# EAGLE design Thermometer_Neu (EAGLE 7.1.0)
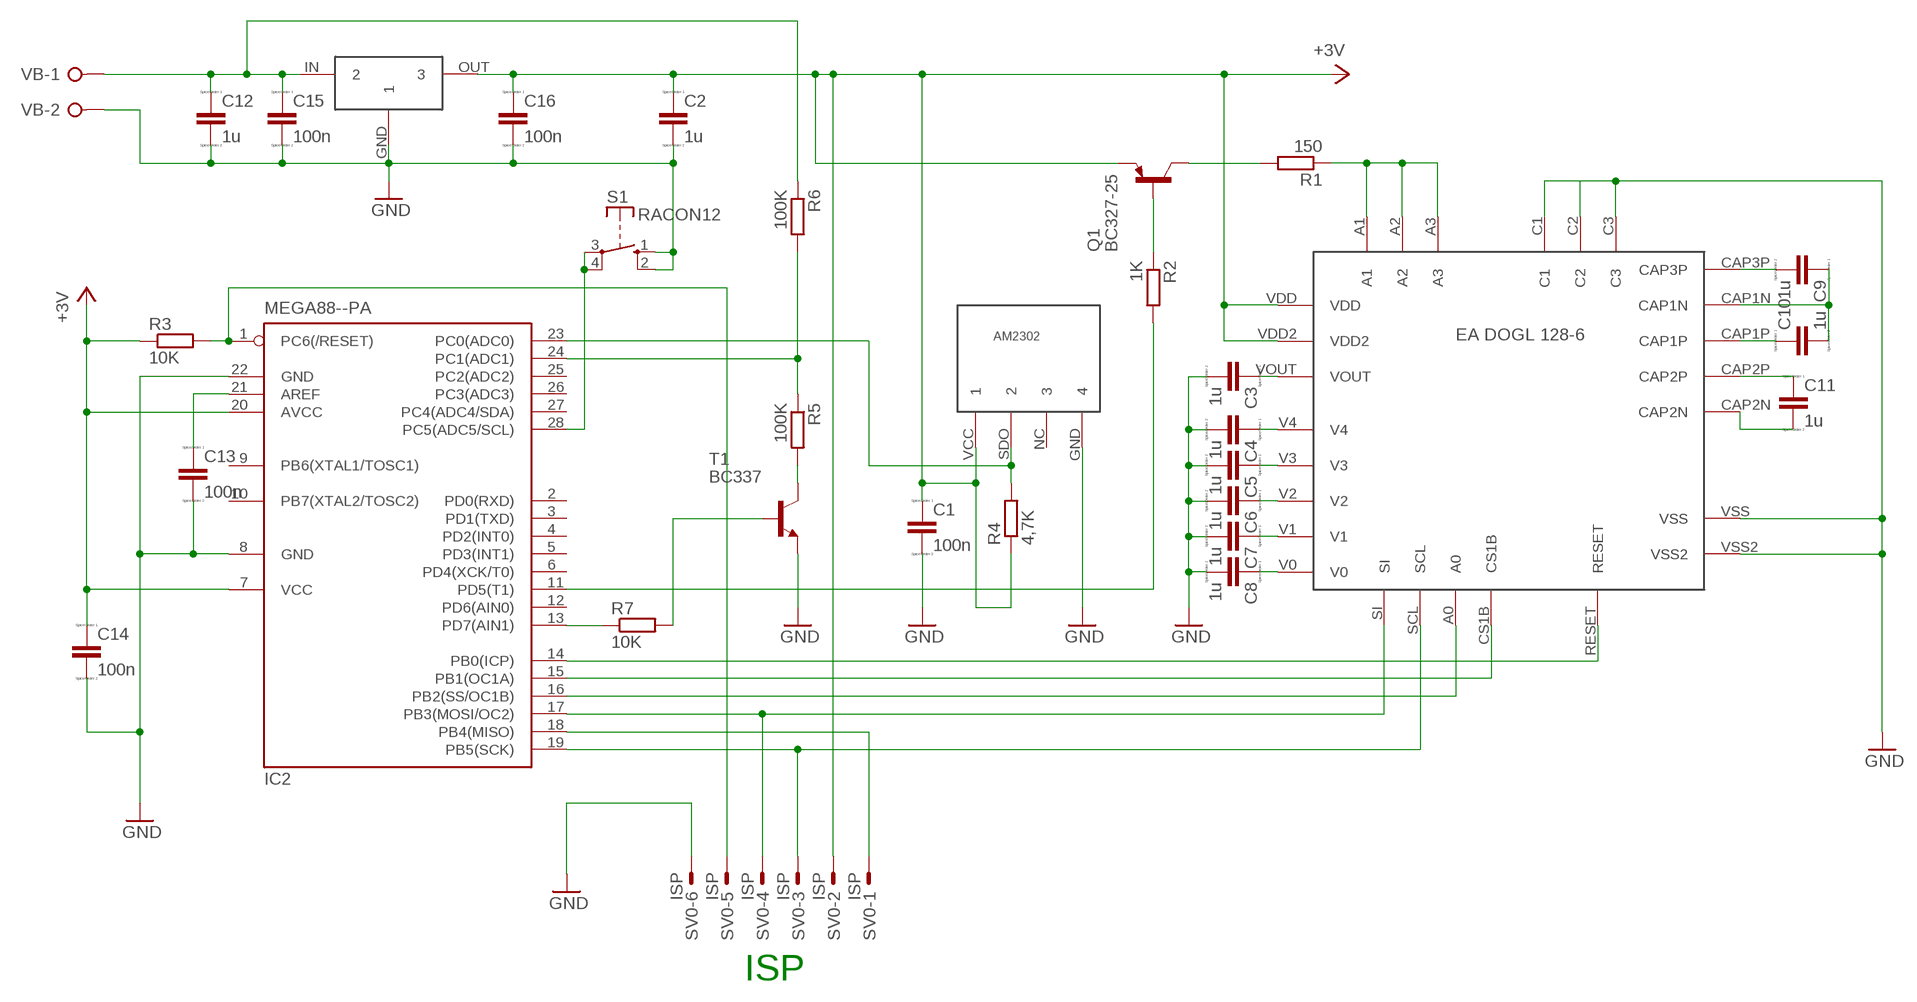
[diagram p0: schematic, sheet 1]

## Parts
C1  100n  C-EUC1206K  [C1206K]
C2  1u  C-EUC1206K  [C1206K]
C3  1u  C-EUC1206K  [C1206K]
C4  1u  C-EUC1206K  [C1206K]
C5  1u  C-EUC1206K  [C1206K]
C6  1u  C-EUC1206K  [C1206K]
C7  1u  C-EUC1206K  [C1206K]
C8  1u  C-EUC1206K  [C1206K]
C9  1u  C-EUC1206K  [C1206K]
C10  1u  C-EUC1206K  [C1206K]
C11  1u  C-EUC1206K  [C1206K]
C12  1u  C-EUC1206K  [C1206K]
C13  100n  C-EUC1206K  [C1206K]
C14  100n  C-EUC1206K  [C1206K]
C15  100n  C-EUC1206K  [C1206K]
C16  100n  C-EUC1206K  [C1206K]
IC2  MEGA88--PA  MEGA8-P  [DIL28-3]
Q1  BC327-25  [TO92-EBC]
R1  150  R-EU_0207/15  [0207/15]
R2  1K  R-EU_0207/15  [0207/15]
R3  10K  R-EU_0207/15  [0207/15]
R4  4,7K  R-EU_0207/15  [0207/15]
R5  100K  R-EU_0207/15  [0207/15]
R6  100K  R-EU_0207/15  [0207/15]
R7  10K  R-EU_0207/15  [0207/15]
S1  RACON12  [RACON12]
SV0  ISP  ML6E  [ML6]
T1  BC337  [TO92]
U$1  LDO  [LDO]
U$2  AM2302  [AM2302]
U$3  EA_DOGL_128_6  [EA_DOGL_128-6]
VB  W237-02P  [W237-132]

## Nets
+3V3: C1.1 C2.1 C14.1 C16.1 IC2.7(VCC) IC2.20(AVCC) Q1.E R3.1 R4.1 SV0.2 U$1.OUT U$2.VCC U$3.VDD U$3.VDD2 ; supply symbol labelled +3V
GND: C1.2 C2.2 C3.2 C4.2 C5.2 C6.2 C7.2 C8.2 C12.2 C13.2 C14.2 C15.2 C16.2 IC2.8(GND) IC2.22(GND) S1.1(S) S1.2(S) SV0.6 T1.1(E) U$1.GND U$2.GND U$3.C1 U$3.C2 U$3.C3 U$3.VSS U$3.VSS2 VB.2
N$1: IC2.19(PB5(SCK)) SV0.3 U$3.SCL
N$2: IC2.17(PB3(MOSI/OC2)) SV0.4 U$3.SI
N$3: IC2.14(PB0(ICP)) U$3.RESET
N$4: IC2.15(PB1(OC1A)) U$3.CS1B
N$5: IC2.16(PB2(SS/OC1B)) U$3.A0
N$6: IC2.18(PB4(MISO)) SV0.1
N$7: C13.1 IC2.21(AREF)
N$8: C3.1 U$3.VOUT
N$9: C4.1 U$3.V4
N$10: R1.1 U$3.A1 U$3.A2 U$3.A3
N$11: Q1.C R1.2
N$12: Q1.B R2.1
N$13: C5.1 U$3.V3
N$14: C6.1 U$3.V2
N$15: C7.1 U$3.V1
N$16: C8.1 U$3.V0
N$17: C9.2 U$3.CAP3P
N$18: C9.1 C10.2 U$3.CAP1N
N$19: C10.1 U$3.CAP1P
N$20: C11.1 U$3.CAP2P
N$21: IC2.11(PD5(T1)) R2.2
N$22: C11.2 U$3.CAP2N
N$24: IC2.1(PC6(/RESET)) R3.2 SV0.5
N$25: C12.1 C15.1 R6.1 U$1.IN VB.1
N$27: IC2.28(PC5(ADC5/SCL)) S1.3(P) S1.4(P)
N$28: IC2.13(PD7(AIN1)) R7.1
N$29: R7.2 T1.2(B)
N$30: R5.2 T1.3(C)
N$31: IC2.24(PC1(ADC1)) R5.1 R6.2
N$32: IC2.23(PC0(ADC0)) R4.2 U$2.SDO
Unconnected: IC2.2(PD0(RXD)) IC2.3(PD1(TXD)) IC2.4(PD2(INT0)) IC2.5(PD3(INT1)) IC2.6(PD4(XCK/T0)) IC2.9(PB6(XTAL1/TOSC1)) IC2.10(PB7(XTAL2/TOSC2)) IC2.12(PD6(AIN0)) IC2.25(PC2(ADC2)) IC2.26(PC3(ADC3)) IC2.27(PC4(ADC4/SDA)) U$2.NC

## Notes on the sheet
- ISP

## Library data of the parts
C1-C16 = resistor:C-EU: CAPACITOR, European symbol; SPICEPREFIX: C
IC2 = atmel:MEGA8-P: MICROCONTROLLER 8 Kbytes FLASH, 1 kbytes SRAM, 512 bytes EEPROM, USART, 4-channel 10 bit ADC, 2-channel 8 bit ADC Pin compatible with Atmega48, ATMega88, ATMega168 Source: avr.lbr; OC_FARNELL: unknown; OC_NEWARK: unknown
Q1 = transistor-pnp:BC327*: PNP Transistror
R1-R7 = resistor:R-EU_: RESISTOR, European symbol
S1 = switch-misc:RACON12: ITT SWITCH
SV0 = con-harting-ml:ML6?E: HARTING; OC_FARNELL: unknown; OC_NEWARK: unknown
T1 = transistor-neu-to92:BC337: NPN TRANSISTOR
U$1 = MCP1702:LDO
U$2 = AM2302:AM2302
U$3 = EA_DOGL_128_6:EA_DOGL_128_6
VB = con-wago-508:W237-02P: WAGO SREW CLAMP; OC_FARNELL: unknown; OC_NEWARK: unknown

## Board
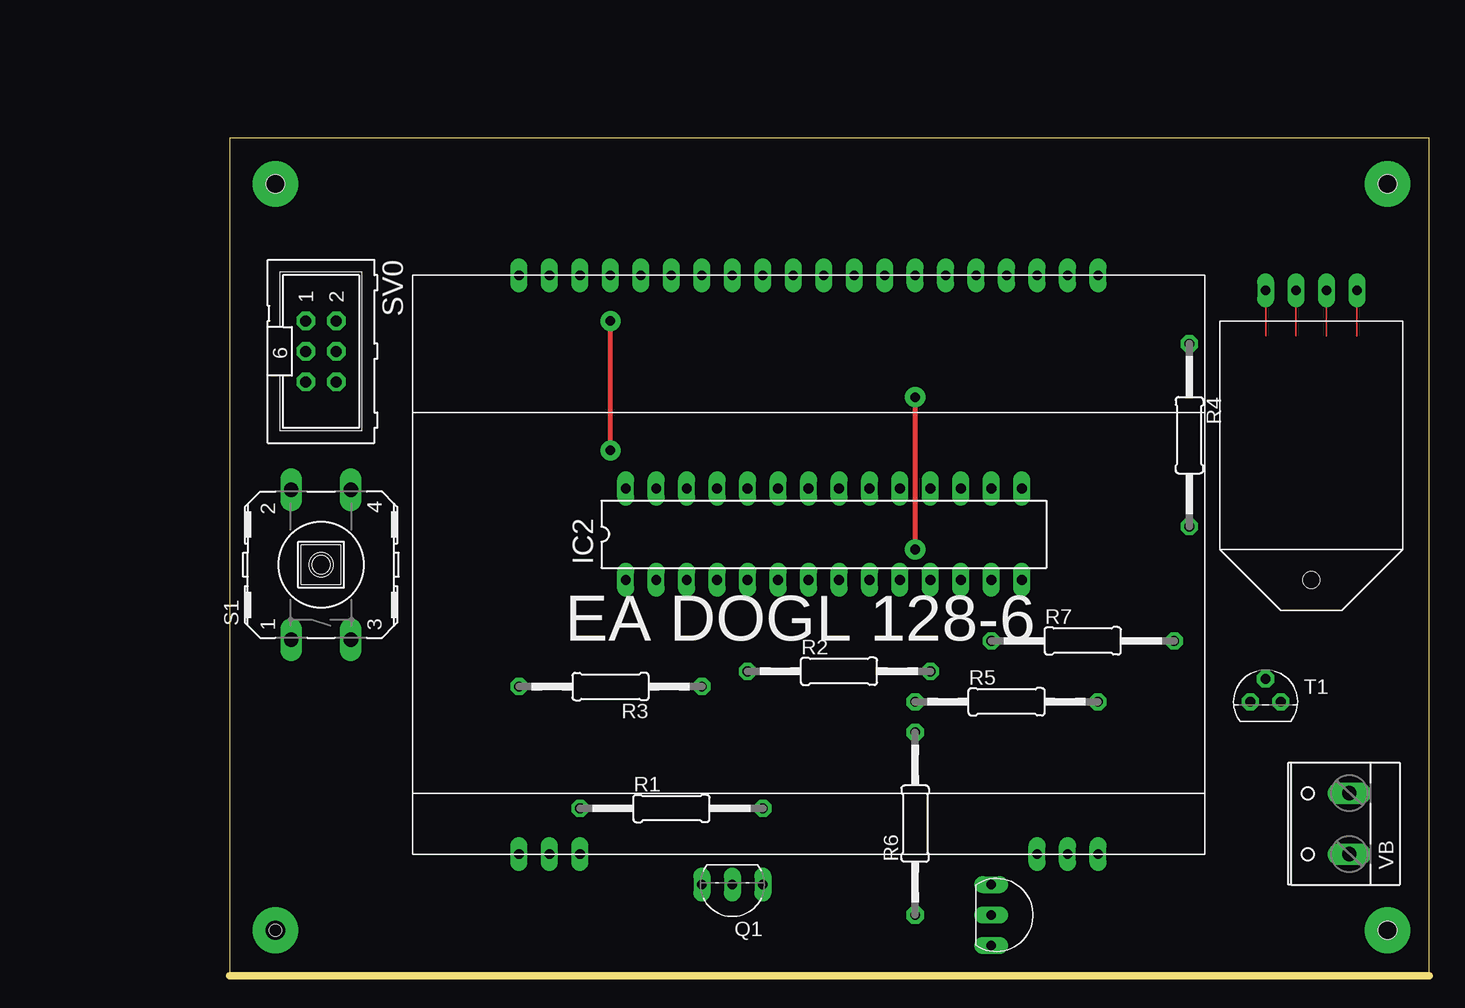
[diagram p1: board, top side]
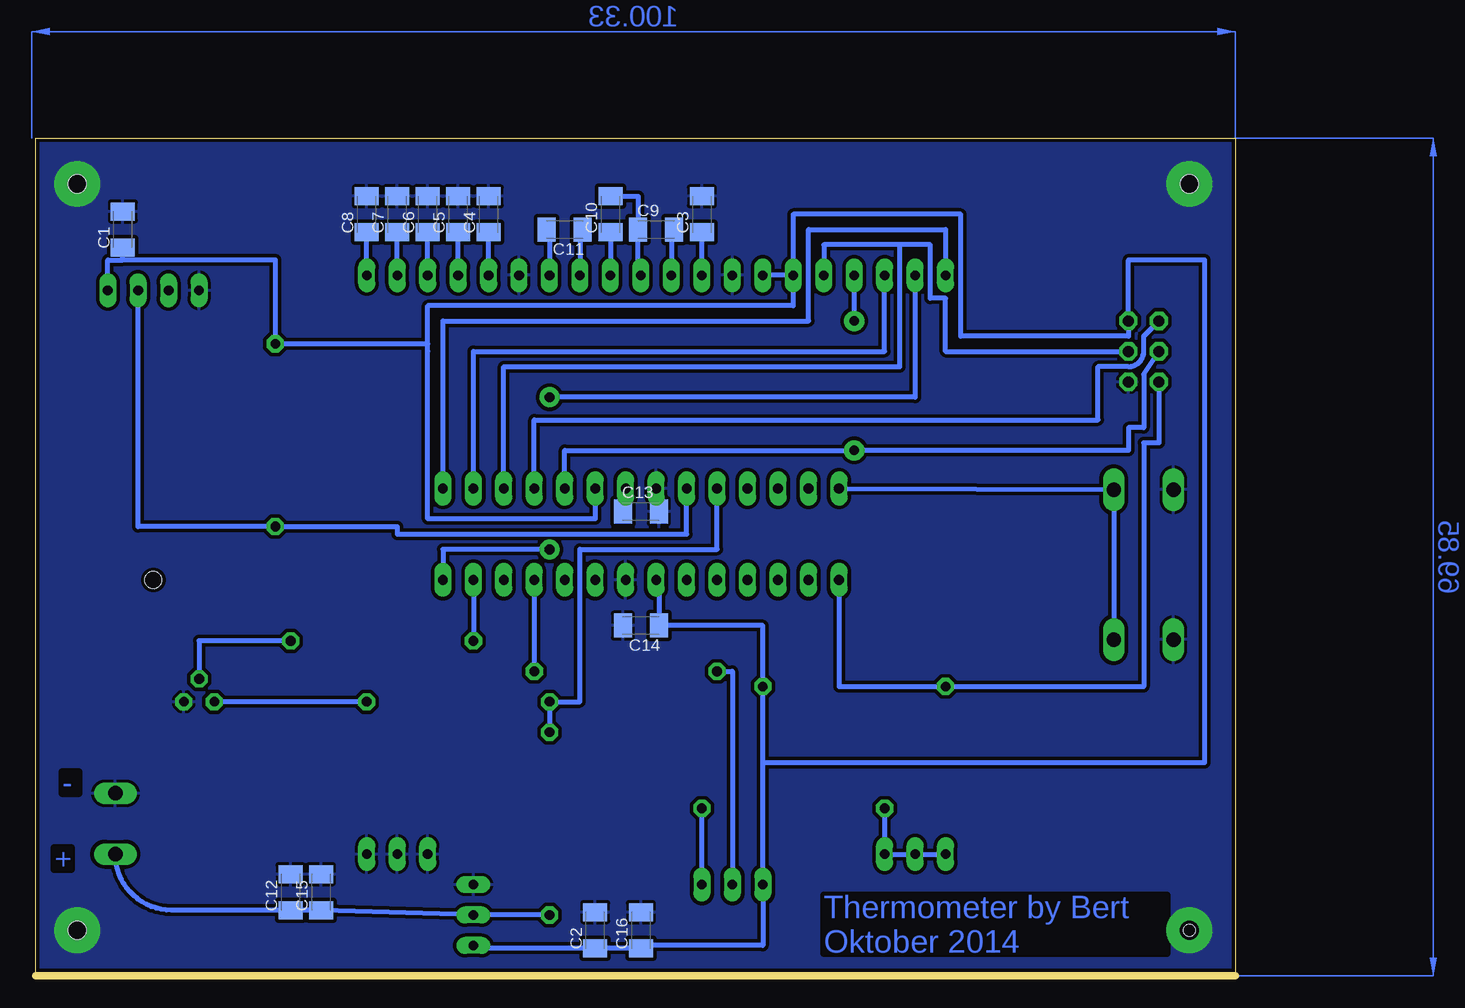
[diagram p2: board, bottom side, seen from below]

Size 100 x 69.84 mm. Coordinates in mm from the lower left corner, seen from the top.
Outline: 0,0 100,0 100,69.84 0,69.84 0,0
Copper layers (1*16): Top 0.035mm / dielectric 1.5mm / Bottom 0.035mm
Design rules "default *": minimum track width 10mil, minimum drill 24mil, track to track 8mil, track to pad 8mil, pad to pad 8mil, via to via 8mil, smd to smd 8mil, copper to edge 10mil, drill to drill 8mil, minimum pad ring 12mil, minimum via ring 12mil, stop-mask expansion 4mil, vias tented up to drill 0mil, thermal gap 10mil
Holes 1.5 mm at 96.52,3.81 96.52,66.04 3.81,66.04
Holes 1 mm at 3.81,3.81

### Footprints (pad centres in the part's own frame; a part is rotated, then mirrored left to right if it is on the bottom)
C1206K = smd 1.5 x 2: 1 -1.5,0; 2 1.5,0
DIL28-3 = drill 0.813 long: 1 -16.51,-3.81; 2 -13.97,-3.81; 3 -11.43,-3.81; 4 -8.89,-3.81; 5 -6.35,-3.81; 6 -3.81,-3.81; 7 -1.27,-3.81; 8 1.27,-3.81; 9 3.81,-3.81; 10 6.35,-3.81; 11 8.89,-3.81; 12 11.43,-3.81; 13 13.97,-3.81; 14 16.51,-3.81; 15 16.51,3.81; 16 13.97,3.81; 17 11.43,3.81; 18 8.89,3.81; 19 6.35,3.81; 20 3.81,3.81; 21 1.27,3.81; 22 -1.27,3.81; 23 -3.81,3.81; 24 -6.35,3.81; 25 -8.89,3.81; 26 -11.43,3.81; 27 -13.97,3.81; 28 -16.51,3.81
TO92-EBC = drill 0.813 long: B 0,-1.27; C -2.54,-1.27; E 2.54,-1.27
0207/15 = drill 0.813 octagon: 1 -7.62,0; 2 7.62,0
RACON12 = drill 1.194 long: 1 -6.248,2.489; 2 6.248,2.489; 3 -6.248,-2.489; 4 6.248,-2.489
ML6 = drill 0.914 octagon: 1 -2.54,-1.27; 2 -2.54,1.27; 3 0,-1.27; 4 0,1.27; 5 2.54,-1.27; 6 2.54,1.27
TO92 = drill 0.813 octagon: 1 1.27,0; 2 0,1.905; 3 -1.27,0
LDO = drill 0.8 long: GND -2.54,-1.27; IN 0,-1.27; OUT 2.54,-1.27
AM2302 = drill 0.8 long: GND 3.81,-11.43; NC 1.27,-11.43; SDO -1.27,-11.43; VCC -3.81,-11.43 | hole 1.4: 0,12.7
EA_DOGL_128-6 = drill 0.8 long: A0 -19.05,25.4; A1 -24.13,-22.86; A2 -21.59,-22.86; A3 -19.05,-22.86; C1 19.05,-22.86; C2 21.59,-22.86; C3 24.13,-22.86; CAP1N 1.27,25.4; CAP1P 3.81,25.4; CAP2N 8.89,25.4; CAP2P 6.35,25.4; CAP3P -1.27,25.4; CS1B -24.13,25.4; RESET -21.59,25.4; SCL -16.51,25.4; SI -13.97,25.4; V0 24.13,25.4; V1 21.59,25.4; V2 19.05,25.4; V3 16.51,25.4; V4 13.97,25.4; VDD -11.43,25.4; VDD2 -8.89,25.4; VOUT -3.81,25.4; VSS 11.43,25.4; VSS2 -6.35,25.4
W237-132 = drill 1.194 long: 1 -2.54,-0.635; 2 2.54,-0.635

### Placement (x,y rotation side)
C1  92.71,62.23 90 bottom
C2  53.34,3.81 90 bottom
C3  44.45,63.5 90 bottom
C4  62.23,63.5 90 bottom
C5  64.77,63.5 90 bottom
C6  67.31,63.5 90 bottom
C7  69.85,63.5 90 bottom
C8  72.39,63.5 90 bottom
C9  48.26,62.23 0 bottom
C10  52.07,63.5 90 bottom
C11  55.88,62.23 180 bottom
C12  78.74,6.99 90 bottom
C13  49.53,38.73 0 bottom
C14  49.53,29.21 180 bottom
C15  76.2,6.99 90 bottom
C16  49.53,3.81 90 bottom
IC2  49.53,36.83 0 top
Q1  41.91,6.35 180 top
R1  36.83,13.97 0 top
R2  50.8,25.4 0 top
R3  31.75,24.13 180 top
R4  80.01,45.09 270 top
R5  64.77,22.86 0 top
R6  57.15,12.7 90 top
R7  71.12,27.94 0 top
S1  7.62,34.29 90 top
SV0  7.62,52.07 270 top
T1  86.36,22.86 0 top
U$1  64.77,5.08 270 top
U$2  90.17,45.72 180 top
U$3  48.26,33.02 0 top
VB  92.71,12.7 90 top

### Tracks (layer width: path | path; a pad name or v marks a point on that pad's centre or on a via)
+3V3
  Bottom 0.2: 67.31,52.7 67.31,52.07
  Bottom 0.406: U$3.VDD U$3.VDD2 | 48.53,33.02 IC2.7 | U$3.VDD 36.83,63.5 22.86,63.5 22.86,53.34 8.89,53.34 SV0.2 8.89,59.69 2.54,59.69 2.54,17.78 39.37,17.78 | 39.37,17.78 Q1.E 39.37,2.54 49.53,2.54 | 39.37,17.78 R3.1 39.37,29.21 C14.1 48.03,33.02 | IC2.20 53.34,38.1 67.31,38.1 67.31,52.07 67.31,55.88 36.83,55.88 U$3.VDD | 67.31,52.7 R4.1 80.01,59.69 92.71,59.69 | C16.1 C2.1 63.5,2.31 | 92.71,59.69 C1.1 | U$2.VCC 93.98,59.69 92.71,59.69
  Bottom 0.61: 49.53,2.54 C16.1 | 63.5,2.31 U$1.OUT | IC2.7 48.03,33.02 | C14.1 48.26,29.21
GND  (via drill 1.6 pad 3.81)
  Bottom 0.305: IC2.22 48.53,40.64
  Bottom 0.406: IC2.8 50.53,33.02
  other vias: 3.81,3.81 3.81,66.04 96.52,66.04 96.52,3.81
  pour Bottom (isolate 0.305): 0,69.85 100.33,69.85 100.33,0 0,0
N$1  (via drill 0.7 pad 1.68, 0.8 pad 1.68)
  Top 0.406: v31.75,43.81 v31.75,54.61
  Bottom 0.406: IC2.19 55.88,43.81 v31.75,43.81 8.89,43.81 8.89,45.72 7.62,45.72 7.62,50.16 SV0.3 | v31.75,54.61 U$3.SCL
N$2
  Bottom 0.406: 27.94,60.96 25.4,60.96 25.4,56.52 24.13,56.52 24.13,52.07 SV0.4 | 27.94,60.96 34.29,60.96 U$3.SI | IC2.17 60.96,50.8 27.94,50.8 27.94,60.96
N$3  (via drill 0.8 pad 1.68)
  Top 0.406: v57.15,48.26 v57.15,35.56
  Bottom 0.406: U$3.RESET 26.67,48.26 v57.15,48.26 | v57.15,35.56 66.04,35.56 IC2.14
N$4
  Bottom 0.406: IC2.15 66.04,54.61 35.56,54.61 35.56,62.23 24.13,62.23 U$3.CS1B
N$5
  Bottom 0.406: IC2.16 63.5,52.07 29.21,52.07 U$3.A0
N$6
  Bottom 0.406: IC2.18 58.42,46.36 11.43,46.36 11.43,50.8 8.89,50.8 arc-90 7.62,52.07 7.62,53.34 SV0.1
N$7
  Bottom 0.406: IC2.21 51.03,40.64 C13.1
N$8
  Bottom 0.406: U$3.VOUT C3.1
N$9
  Bottom 0.406: U$3.V4 C4.1
N$10
  Bottom 0.406: R1.1 U$3.A3 U$3.A2 U$3.A1
N$11
  Bottom 0.406: Q1.C R1.2
N$12
  Bottom 0.406: R2.1 41.91,25.4 Q1.B
N$13
  Bottom 0.406: U$3.V3 C5.1
N$14
  Bottom 0.406: U$3.V2 C6.1
N$15
  Bottom 0.406: U$3.V1 C7.1
N$16
  Bottom 0.406: U$3.V0 C8.1
N$17
  Bottom 0.406: 46.76,58.42 U$3.CAP3P 46.99,62.23 C9.2
N$18
  Bottom 0.406: U$3.CAP1N 49.76,58.42 C9.1 49.76,65 C10.2
N$19
  Bottom 0.406: C10.1 U$3.CAP1P
N$20
  Bottom 0.406: 54.88,58.42 U$3.CAP2P 54.61,62.23 C11.1
N$21
  Bottom 0.406: IC2.11 R2.2
N$22
  Bottom 0.406: 56.88,58.42 U$3.CAP2N 57.15,62.23 C11.2
N$24
  Bottom 0.406: SV0.5 6.35,44.45 7.62,44.45 7.62,24.13 R3.2 33.02,24.13 IC2.1
N$25
  Bottom 0.406: R6.1 U$1.IN C15.1 C12.1 88.67,5.49 arc90 VB.1
N$27
  Bottom 0.406: IC2.28 S1.4 S1.3
N$28
  Bottom 0.406: IC2.13 R7.1
N$29
  Bottom 0.406: T1.2 86.36,27.94 R7.2
N$30
  Bottom 0.406: R5.2 T1.3
N$31
  Bottom 0.406: 43.18,39.37 IC2.24 43.18,35.56 54.61,35.56 54.61,22.86 R5.1 R6.2
N$32
  Bottom 0.406: U$2.SDO 91.44,37.47 R4.2 69.85,37.47 69.85,36.83 45.72,36.83 IC2.23
(copper drawn outside any net)
  shapes: Bottom area x2

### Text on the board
Bottom: - | + | Thermometer by Bert / Oktober 2014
